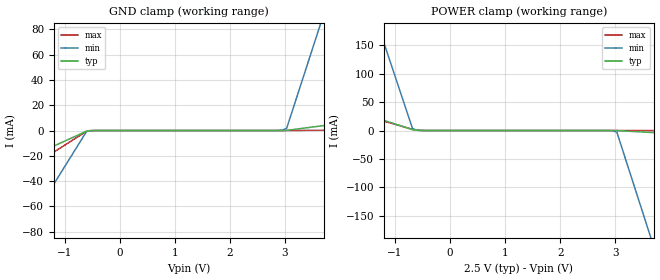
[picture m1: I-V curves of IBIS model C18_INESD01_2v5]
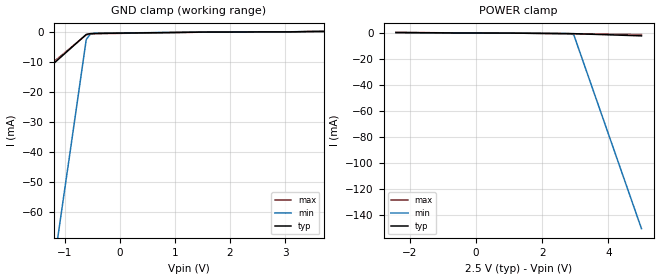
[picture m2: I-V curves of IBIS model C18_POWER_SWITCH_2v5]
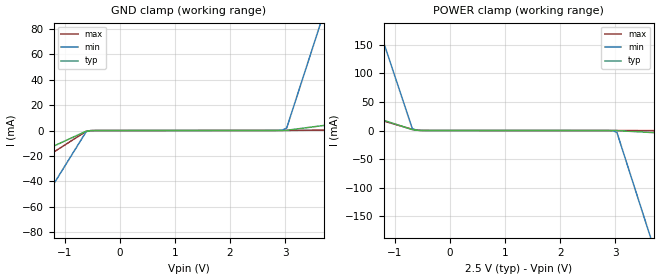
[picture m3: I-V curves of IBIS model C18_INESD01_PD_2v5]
|   This file is an IBIS representation of the   |
|   Integrated Device Technology , Inc.   |
|   8N3QV01   |
|   Quad-Frequency Programmable VCXO   |
[IBIS Ver]   4.1
[File name]   8n3qv01.ibs
[File Rev]   1.0
[Date]   20 Aug 2009 | Last modified
[Source]   Originated at Integrated Device Technology, Inc.
[Disclaimer]
IDT hereby grants the user of this IBIS model a non-exclusive,
nontransferable license to use this IBIS model under the following terms.
Before using this IBIS model, the user should read this license.
If the user does not accept these terms,  the IBIS model should be
returned to IDT within 30 days.
   The user is granted this license only to use the IBIS model and
is not granted rights to sell, load, rent, lease or license the IBIS
model in whole or in part, or in modified form to anyone other than
user. User may modify the IBIS model to suit its specific
applications but rights to derivative works and such modifications
shall belong to IDT.
   This IBIS model is provided on an "AS IS" basis and IDT makes
absolutely no warranty with respect to the information contained
herein. IDT DISCLAIMS AND CUSTOMER WAIVES ALL WARRANTIES, EXPRESS
OR IMPLIED, INCLUDING WARRANTIES OF MERCHANTABILITY OR FITNESS FOR
A PARTICULAR PURPOSE. The entire risk as to quality and performance
is with the Customer. ACCORDINGLY, IN NO EVENT SHALL THE COMPANY BE
LIABLE FOR ANY DAMAGES, WHETHER IN CONTRACT OR TORT,INCLUDING ANY
LOST PROFITS OR OTHER INCIDENTAL, CONSEQUENTIAL, EXEMPLARY, OR
PUNITIVE DAMAGES ARISING OUT OF THE USE OR APPLICATION OF THE IBIS
model provided in this package. Further, IDT reserves the right to
make changes without notice to any product herein to improve
reliability, function, or design. IDT does not convey any license
under patent rights or any other intellectual property rights,
including those of third parties.
   IDT is not obligated to provide maintenance or support
for the licensed IBIS model.
[Copyright]   Copyright 2009 by Integrated Device Technology , Inc.
[Component]   8N3QV01
[Manufacturer] Integrated Device Technology, Inc.
[Package]
|10 Lead 5x7 Ceramic
|   Typ   Min   Max
R_pkg   58.62m  34.57m  83.84m
L_pkg   1.0618n 0.429n  1.726n
C_pkg   0.236p  0.143p  0.333p
[Pin]   signal_name   model_name   R_pin   L_pin   C_pin
1   VC   C18_INESD01   47.43m  0.767n  0.192p
2   OE   C18_POWER_SWITCH   57.03m  1.020n  0.229p
3   GND   GND   56.57m  1.008n  0.228p
4   FSEL0   C18_INESD01_PD   55.33m  0.975n  0.223p
5   FSEL1   C18_INESD01_PD_I   34.57m  0.428n  0.143p
6   Q   C18_OHSPECL05_OE   53.78m  0.934n  0.217p
7   nQ   C18_OHSPECL05_OE   54.71m  0.959n  0.221p
8   VCC   POWER   71.29m  1.395n  0.284p
9   SDATA   C18_I2C_SDATA_IO   83.84m  1.725n  0.333p
10   SCLK   C18_INESD01_PU   71.60m  1.403n  0.286p
[Diff Pin]   inv_pin   vdiff   tdelay_typ   tdelay_min   tdelay_max
6   7   NA   0   0   0
[Model Selector] C18_INESD01
C18_INESD01_2v5  Buffer selection for 2v5
C18_INESD01_3v3  Buffer selection for 3v3
[Model Selector] C18_POWER_SWITCH
C18_POWER_SWITCH_2v5  Buffer selection for 2v5
C18_POWER_SWITCH_3v3  Buffer selection for 3v3
[Model Selector] C18_INESD01_PD
C18_INESD01_PD_2v5  Buffer selection for 2v5
C18_INESD01_PD_3v3  Buffer selection for 3v3
[Model Selector] C18_INESD01_PD_I
C18_INESD01_PD_I_2v5  Buffer selection for 2v5
C18_INESD01_PD_I_3v3  Buffer selection for 3v3
[Model Selector] C18_OHSPECL05_OE
C18_OHSPECL05_OE_2v5  Buffer selection for 2v5
C18_OHSPECL05_OE_3v3  Buffer selection for 3v3
[Model Selector] C18_I2C_SDATA_IO
C18_I2C_SDATA_IO_2v5  Buffer selection for 2v5
C18_I2C_SDATA_IO_3v3  Buffer selection for 3v3
[Model Selector] C18_INESD01_PU
C18_INESD01_PU_2v5  Buffer selection for 2v5
C18_INESD01_PU_3v3  Buffer selection for 3v3
| Models and submodels in the file (14): C18_INESD01_2v5 (Input), C18_POWER_SWITCH_2v5 (Input), C18_INESD01_PD_2v5 (Input), C18_INESD01_PD_I_2v5 (Input), C18_OHSPECL05_OE_2v5 (Output_ECL), C18_I2C_SDATA_IO_2v5 (Input), C18_INESD01_PU_2v5 (Input), C18_INESD01_3v3 (Input), C18_POWER_SWITCH_3v3 (Input), C18_INESD01_PD_3v3 (Input), C18_INESD01_PD_I_3v3 (Input), C18_OHSPECL05_OE_3v3 (Output_ECL), C18_I2C_SDATA_IO_3v3 (Input), C18_INESD01_PU_3v3 (Input)
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[Model] C18_INESD01_2v5
Model_type   Input
Polarity   Non-Inverting
Vinl = 0.7V
Vinh = 1.7V
|   typ   min   max
C_comp   2pF   1.5pF   2.5pF
|   typ   min   max
[Voltage range]   2.5V   2.375V   2.625V
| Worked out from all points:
|   GND clamp passes 1 mA (typ) near -0.63 V on its own axis
|   POWER clamp passes 1 mA (typ) near -0.64 V on its own axis
[GND_clamp]
|Voltage   I (typ)   I (min)   I (max)
-2.5V     -38.14mA   -133.3mA   -53.19mA
-1.818V   -24.59mA   -85.6mA    -34.25mA
-1.742V   -23.08mA   -80.3mA    -32.15mA
-606.1mV  -499.4uA   -801.4uA   -592uA
-454.5mV  -14.2uA    -20.82uA   -8.773uA
2.955V    16.44uA    367.9uA    89.29nA
3.03V     116.5uA    1.826mA    2.018uA
3.561V    3.108mA    73.05mA    183.6uA
3.636V    3.536mA    83.23mA    209.5uA
5V        11.23mA    266.4mA    676.4uA
[Power_clamp]
|Voltage   I (typ)   I (min)   I (max)
-2.5V     58.41mA    531.6mA    53.28mA
-1.364V   22.9mA     201.5mA    21.24mA
-1.288V   20.54mA    179.5mA    19.11mA
-681.8mV  1.596mA    3.368mA    2.023mA
-606.1mV  543.9uA    639.7uA    668.1uA
-454.5mV  16.44uA    21.47uA    11.81uA
2.955V    -14.2uA    -412.7uA   -82.31nA
3.03V     -94.87uA   -2.923mA   -1.544uA
3.561V    -2.927mA   -162.8mA   -136uA
3.636V    -3.331mA   -185.6mA   -155.2uA
5V        -10.61mA   -596.7mA   -500.8uA
[Model] C18_POWER_SWITCH_2v5
Model_type   Input
Polarity   Non-Inverting
Vinl = 0.7V
Vinh = 1.7V
|   typ   min   max
C_comp   2pF   1.5pF   2.5pF
|   typ   min   max
[Voltage range]   2.5V   2.375V   2.625V
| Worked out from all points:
|   GND clamp passes 1 mA (typ) near -0.62 V on its own axis
[GND_clamp]
|Voltage   I (typ)   I (min)   I (max)
-2.424V   -30.6mA    -235mA     -28.61mA
-1.136V   -9.493mA   -70.29mA   -9.004mA
-1.061V   -8.251mA   -60.6mA    -7.851mA
-606.1mV  -801.2uA   -2.477mA   -932.4uA
-530.3mV  -539.6uA   -666.5uA   -636.9uA
-378.8mV  -453.7uA   -388.8uA   -548.2uA
1.364V    -69.12uA   -22.74uA   -85.15uA
5V        417.6uA    364.3uA    500.2uA
[Power_clamp]
|Voltage   I (typ)   I (min)   I (max)
-2.424V   404.7uA    335.7uA    510.7uA
2.727V    -419.4uA   -382uA     -474.1uA
2.879V    -453.7uA   -526uA     -514.5uA
2.955V    -477.4uA   -1.442mA   -534.8uA
5V        -2.158mA   -150.8mA   -1.103mA
[Model] C18_INESD01_PD_2v5
Model_type   Input
Polarity   Non-Inverting
Vinl = 0.7V
Vinh = 1.7V
|   typ   min   max
C_comp   2pF   1.5pF   2.5pF
|   typ   min   max
[Voltage range]   2.5V   2.375V   2.625V
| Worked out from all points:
|   GND clamp passes 1 mA (typ) near -0.63 V on its own axis
|   POWER clamp passes 1 mA (typ) near -0.63 V on its own axis
[GND_clamp]
|Voltage   I (typ)   I (min)   I (max)
-2.5V     -38.19mA   -133.3mA   -53.24mA
-1.818V   -24.63mA   -85.64mA   -34.29mA
-1.742V   -23.12mA   -80.33mA   -32.19mA
-606.1mV  -511.5uA   -812.7uA   -604.9uA
-454.5mV  -23.28uA   -29.32uA   -18.42uA
2.955V    75.5uA     423.2uA    62.82uA
3.03V     177.1uA    1.883mA    66.35uA
3.561V    3.18mA     73.12mA    259.2uA
3.636V    3.609mA    83.3mA     286.7uA
5V        11.33mA    266.5mA    782.6uA
[Power_clamp]
|Voltage   I (typ)   I (min)   I (max)
-2.5V     58.51mA    531.7mA    53.39mA
-1.364V   22.98mA    201.5mA    21.33mA
-1.288V   20.61mA    179.5mA    19.19mA
-681.8mV  1.659mA    3.425mA    2.094mA
-606.1mV  606uA      695.4uA    736.7uA
-454.5mV  75.5uA     74.38uA    77.19uA
2.955V    -23.28uA   -423.5uA   -7.079uA
3.03V     -105.5uA   -2.935mA   -10.15uA
3.561V    -2.948mA   -162.8mA   -155.8uA
3.636V    -3.354mA   -185.7mA   -176.6uA
5V        -10.66mA   -596.8mA   -551.3uA
